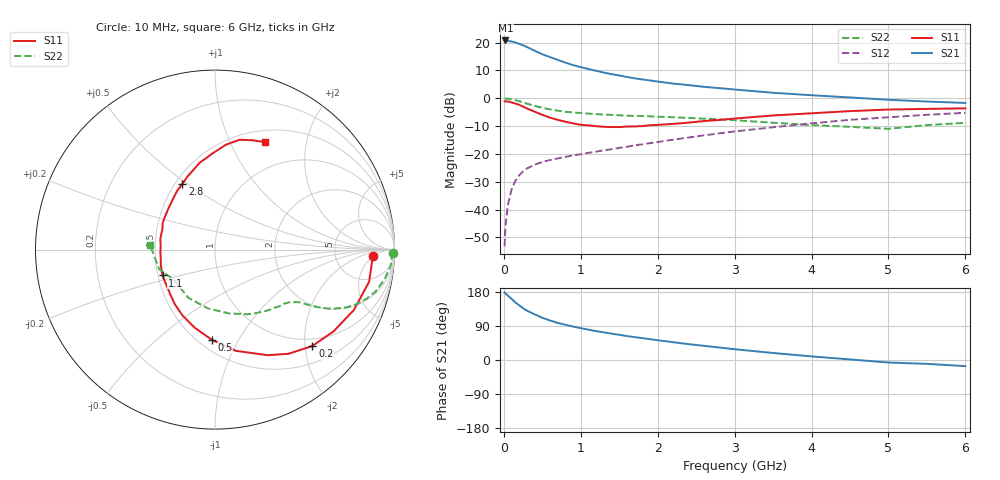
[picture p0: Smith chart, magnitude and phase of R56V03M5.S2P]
! SIEMENS Small Signal Semiconductors
! BFR183
! Si NPN RF Bipolar Junction Transistor in SOT23
! VCE = 6 V  IC = 3.5 mA
! Common Emitter S-Parameters:  May  1996
# GHz  S  MA  R  50
!  f  S11  S21  S12  S22
! GHz  MAG  ANG  MAG  ANG  MAG  ANG  MAG  ANG
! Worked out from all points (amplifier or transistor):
!   36 points, 10 MHz to 6 GHz, reference 50 ohm
!   highest |S21| = 20.8 dB at 20 MHz (marker M1)
!   |S21| within 3 dB of that: start of sweep to 348.7 MHz
!   unconditionally stable (mu >= 1): 1.22 GHz to 2.753 GHz
!   at 250 MHz: K = 0.32, MSG = 22.6 dB, |S12| = -26.2 dB
!   at 1.4 GHz: K = 1.05, MAG = 12.1 dB, |S12| = -18.3 dB
!   at 6 GHz: K = 0.88, MSG = 1.8 dB, |S12| = -5.2 dB
!   S11 on the Smith chart (normalised r, x): 10 MHz: 14, -5; 200 MHz: 0.84, -2.16; 500 MHz: 0.58, -0.78; 1.1 GHz: 0.53, -0.17; 2.8 GHz: 0.54, +0.48; 6 GHz: 0.64, +1.36
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0.01  0.8806 -2.4  10.82 178.2  0.0022 92.4  0.9924 -1.0
0.02  0.8773 -4.7  10.95 175.9  0.0048 83.7  0.9859 -2.1
0.05  0.8771 -11.8  10.77 170.4  0.0116 82.0  0.983 -5.3
0.1  0.8437 -23.5  10.51 161.4  0.023 78.3  0.9584 -10.1
0.15  0.8028 -34.5  10.08 151.8  0.0328 71.5  0.9243 -14.7
0.2  0.7633 -44.7  9.499 144.2  0.0414 67.4  0.8859 -18.1
0.25  0.7103 -54.8  8.945 136.8  0.0487 63.0  0.8432 -21.2
0.3  0.6574 -63.5  8.348 130.2  0.0548 60.3  0.8006 -23.7
0.4  0.5757 -78.4  7.163 120.5  0.0643 55.9  0.7293 -26.9
0.5  0.5036 -91.9  6.182 111.5  0.0718 53.2  0.6756 -28.7
0.6  0.4492 -104.7  5.496 104.2  0.0776 52.0  0.6321 -29.9
0.7  0.41 -116.0  4.899 98.1  0.0829 51.4  0.5991 -30.8
0.9  0.3538 -134.5  3.946 88.3  0.0942 51.5  0.5558 -31.9
1.1  0.3258 -153.8  3.356 80.1  0.1047 52.4  0.5305 -33.5
1.4  0.3045 -177.6  2.711 69.5  0.1214 54.5  0.5025 -36.1
1.6  0.3108 168.7  2.418 63.2  0.1347 55.3  0.4874 -38.2
2.2  0.3463 138.5  1.839 47.0  0.1804 56.0  0.4562 -46.8
2.8  0.4082 116.4  1.521 33.0  0.2339 53.6  0.4175 -58.4
3.5  0.4913 100.0  1.256 18.5  0.3014 47.5  0.3636 -77.8
4.5  0.588 84.0  1.035 1.5  0.4104 36.4  0.307 -119.0
5.5  0.6445 70.9  0.874 -10.2  0.5051 23.4  0.3297 -160.4
6  0.6599 65.2  0.825 -16.2  0.5488 15.0  0.3619 176.3
